//05.04.99
//Umstrukturierung, Aufruf FB2 mit Multiinstanz-DB
//Lesen von numMagPlaceParam bei Neustart da Änderung Anzahl Par. in SW 5 (8)
//DB92 - DB94 entfallen da Aufruf FB2 mit Multiiinstanz-DB
//neue Fkt: TNr_write=1, Vorgabe TNummer in TNr_FB2 von extern
//


FUNCTION_BLOCK FB 91
TITLE = LE_SUCH
// Fehler-Nr. in Ausgangsparameter State:
// 1 = Fehler FB2 interne T-Nummer lesen
// 2 = Kein Werkzeug in LocNr_ZW vorhanden
// 3 = Fehler FB4 PI-Dienst TMFDPL
// 4 = Fehler FB2 Rückgabeparameter lesen
// 5 = Leerplatzsucheauftrag mit Fehler beendet
//     Rückmeldung PI-Dienst von Variablen
// 6 = Schrittnummer unzulaessig
// 7 = Fehler Variable numPlaceParams lesen
//     -> Neustart erforderlich
// 8 = Fehler FB4 PI-Dienst MMCSEM
VERSION : 2.0

VAR_INPUT
    Start: Bool; // Start Leerplatz suchen für WZ in Zwischensp. mit pos.Flanke
    MagNr_ZW: Int; // Magazin-Nr. Zwischenspeicher
    LocNr_ZW: Int; // Platz-Nr. Zwischenspeicher
    MagNr: Int; // Magazin-Nr. der Leerplatzsuche
END_VAR

VAR_OUTPUT
    Activ:	Bool; // Baustein aktiv, Leerplatzsuche läuft
    Done: Bool; // Leerplatz gefunden
    Error: Bool; // Fehler
    State: Word; // Fehler-Nummer
    MagNr_Empty: Int; // Magazin-Nr. Leerplatz
    LocNr_Empty: Int; // Platz-Nr. Leerplatz
END_VAR

VAR
    TOANr: Byte:=b#16#1; // TOA-Bereich
    TNr_FB2: Int; // T-Nummer Magazinplatz
    TNr_write: Bool:=False; // Status=1:T-Nummer von Anwender versorgt
    MMCSEM: Bool:=False; // Status=1:Semaphoren nicht setzen
    numMagPlaceParams: Word; // Anzahl Parameter eines Magzinplatzes
    numPlacePar_read: Bool; //Variable nummagplaceparams lesen nach Neustart
    numPlacePar_Error: Bool; // Fehler bei Variable nummagplaceparams lesen
    numPlacePar_ok: Bool; // Variable numMagPlaceParams gelesen ohne Fehler
    HM_Fehler: Bool;
    Schrittregister : BYTE ;
    StateFB2_TNrGesp: Word; // Ausgang State FB2 T-Nr. lesen gespeichert
    StateFB2_ParGesp: Word; // Ausgang State FB2 Parameter lesen gespeichert
    StateFB4_Gesp:Word; // Ausgang State FB4 PI-Dienst Leerplatz suchen gespeichert
    BeZustdMag: Word; // Bereich Befehlszustand des Magazins bei Par. lesen
    MagNrLeerplatz: Word; // Bereich Magazin-Nummer Leerplatz bei Par.lesen
    PlNrLeerplatz: Word; // Bereich Platz-Nummer Leerplatz bei Par. lesen
    Value: Word; // Semaphore Value
    Zaehler: Int; // Zähler für Zeitüberwachung State 3 bei
    GET_FB2 : FB 2;
    PI_Dienste_FB4 : FB 4;
END_VAR
VAR_TEMP
    Error_FB2: Bool; // Error FB2
    NDR_FB2: Bool; // Auftrag beendet FB2
    Error_FB4: Bool; // Error FB4
    Done_FB4: Bool; // Auftrag beendet FB4
    LocLine: Word; // Zeilenadresse Log. T-Nr. lesen
    Column_FB2: Word; // Spaltenadresse FB2
    State_FB2: Word; // Fehler-Nr. FB2 T-Nr. lesen
    State_FB4: Word; // Fehler-Nr. FB4
    TOA: Int; // Eingang Unit FB4 PI-Dienst Leerplatz suchen
    TNr: Word; // Eingang WVar1 FB4 PI-Dienst Leerplatz suchen
    PlNrWohin: Word; // Eingang WVar2 FB4 PI-Dienst Leerplatz suchen
    MagNrWohin: Word; // Eingang WVar3 FB4 PI-Dienst Leerplatz suchen
    PlNr_Bez:  Word; // Eingang WVar4 FB4 PI-Dienst Leerplats suchen
    MagNr_Bez: Word; // Eingang WVar5 FB4 PI-Dienst Leerplats suchen
END_VAR

BEGIN
     UN	DB8.DBX45.0;
     SPB 	ANF1;		// Neustart ? Nein ->
     CALL	#GET_FB2 (
      	Req				:= FALSE);
     CALL	#PI_Dienste_FB4  (
		Req				:= FALSE);
	SET;
      R	numPlacePar_Error;
 	S	numPlacePar_read;
	R      numPlacePar_ok;
	SPA	LOEP;
ANF1:UN	numPlacePar_read;
     SPB	ANF2;
     call #GET_FB2 ( // -- Anzahl Parameter eines Magazinplatz lesen --
     Req:=TRUE, // Variable lesen
     NumVar:= 1, // Anzahl der zu lesenden Variablen
     Addr1:=WZV_VAR.N_Y_numMagPlaceParams_27, // Variable numMagPlaceParams
     Error:=#Error_FB2, // NC_VAR lesen beendet mit Fehler
     NDR:=#NDR_FB2, // NC_VAR lesen beendet ohne Fehler
     State:=#State_FB2, // Fehler-Nummer bei Error = 1
     RD1:=numMagPlaceParams); // Wert in numMagPlaceParams
     UN    #NDR_FB2; // Lesen beendet ohne Fehler
     UN    #Error_FB2; // Lesen beendet mit Fehler
     SPB   ENDE; // Lesen beendet ? Nein ->
     call #GET_FB2 ( // FB2 freigeben
     Req:=False);
     UN    #Error_FB2;
     R     numPlacePar_read;
     S     numPlacePar_ok;
     SPB   ENDE; // Lesen beendet mit Fehler ? Nein ->
     L     6;
     L     #State_FB2;
     ==I;
     SPB   ENDE; // FIFO voll -> Lesen wiederholen
     S     numPlacePar_Error;
     R     numPlacePar_read;
     T     StateFB2_TNrGesp; // Fehlernummer speichern
     SPA   ENDE;
ANF2:U   Start;
     SPB ANF;
LOEP:R    Done; // Ausgangsparameter Done nur 1 PLC-Zyklus
     R    Error; // Ausgangsparameter Error nur 1 PLC-Zyklus
     R    Activ;
     L    0;
     T    State; // Fehler-Nr. = 0
     SPA  ENDE;
ANF: U    Activ;
     SPB  SPRG; // Baustein aktiv ? Ja ->
     U   numPlacePar_Error;
     ON  numPlacePar_ok;
     L	7;
     SPB  FEHL; // Fehler bei Variable numMagPlaceParams lesen ->
     S    Activ; // Hilfsvariable vorbesetzen
     R    Done;
     R    Error;
     R    HM_Fehler;
     L    0;
     T    Zaehler;
     T    State; // Fehler-Nr. = 0
     T    MagNr_Empty;
     T    LocNr_Empty;
     T    Schrittregister;
SPRG:L    Schrittregister;
     SPL  FEHS; // Sprungverteiler
     SPA  SR1; // T-Nr. lesen
     SPA  SR2; // Semaphore setzen
     SPA  SR3; // Start PI-Dienst Leerplatz suchen
     SPA  SR4; // Rückgabeparameter lesen
     SPA  SR5; // Semaphore freigeben
FEHS:L 6;
     SPA  FEHL;
SR1: U    TNr_write;
     SPB  QFEH; // T-Nummer von Anwender -> keine TNr lesen
     L    MagNr_ZW; // ----Schritt 1: T-Nr. lesen --------------------
     T    Column_FB2; // Spalte Addr1 = Magazin-Nummer
     L    LocNr_ZW; // Platz-Nr. Zwischenspeicher
     +    -1;
     L    numMagPlaceParams; // Anzahl Parameter pro MagPlatz
     *I; // (PlatzNr.-1)*numMagPlaceParams+Parameter-Nr.
     +    3;
      T #LocLine; // Zeile Addr1 = T-Nr. von Platz 3
     call #GET_FB2 ( // -- Magazinplatzdaten lesen --
     Req:=TRUE, // Variable lesen
     NumVar:= 1, // Anzahl der zu lesenden Variablen
     Addr1:=WZV_VAR.T0_TP_placeData0_0, // T-Nummer von WZ in Zwischenspeicher
     Unit1:=TOANr, // Bereich = TOA 1
     Line1:=#LocLine, // Zeilenadresse
     Column1:=#Column_FB2, // Spaltenadresse
     Error:=#Error_FB2, // NC_VAR lesen beendet mit Fehler
     NDR:=#NDR_FB2, // NC_VAR lesen beendet ohne Fehler
     State:=#State_FB2, // Fehler-Nummer bei Error = 1
     RD1:=TNr_FB2); // Zielbereich für T-Nummer = TNr_FB2
     UN    #NDR_FB2; // Lesen beendet ohne Fehler
     UN    #Error_FB2; // Lesen beendet mit Fehler
     SPB   ENDE; // Lesen beendet ? Nein ->
     call #GET_FB2 ( // FB2 freigeben
     Req:=False);
     UN    #Error_FB2;
     SPB   QFEH; // Lesen beendet mit Fehler ? Nein ->
     L	6;
     L	#State_FB2;
     ==I;
     SPB	ENDE;
     T StateFB2_TNrGesp; // Fehlernummer speichern
     L     1; // Fehler-Nummer FB 91 = 1
     SPA   FEHL;
QFEH:L     TNr_FB2;	// logische T-Nummer von WZ in Zwischenspeicher
     L     0;
     ==I;
     L     2;
     SPB   FEHL; // T-Nr. in Zwischensp. = 0 ? -> Kein Leerplatz suchen
     U     MMCSEM;
     SPB  SR3A; // Semaphoren nicht setzen ->
     L     1;
     T     Schrittregister;
     T     Value;
SR2: L     TOANr;
     T     #TOA;
     CAll  #PI_Dienste_FB4 ( // -- PI-Dienst Semaphoren starten --
     Req:=TRUE, // Start PI-Dienst
     PIService:=PI.MMCSEM, // PI-Dienst Leerplatz suchen
     Unit:=#TOA, // TO-Nummer
     WVar1:=w#16#2, // FunctionNumber =2
     WVar2:=Value, // Semaphore Value
     Error:=#Error_FB4,
     Done:=#Done_FB4,
     State:=#State_FB4);
     UN    #Error_FB4;
     UN    #Done_FB4;
     SPB   ENDE;	// Leerplatzsuche beendet ? Nein ->
     CALL #PI_Dienste_FB4 ( // -- PI-Dienst Leerplatz suchen  beenden --
     Req:=False); // Start PI-Dienst
     UN    #Error_FB4;
     SPB   QFE1; // Leerplatzsuche beendet mit Fehler ? Nein ->
     L     #State_FB4;
     T     StateFB4_Gesp; // Fehler-Nummer FB 4 speichern
     L     3;
     <>I;
     L     8; // Fehler-Nummer FB 91 = 8
     SPB   FEHL;
     L     1;
     L     Schrittregister;
     <>I;
     L     8;
     SPB   FEHL; // Fehler bei Abwahl Semaphore
     L     Zaehler;
     +     1;
     T     Zaehler;
     L     300;
     >=I;
     L     8;
     SPB   FEHL; // Wartezeit ´überschritten ->
     SPA   ENDE; // Semaphore setzen wiederholen bis kein Fehler kommt
QFE1:U     HM_Fehler;
     SPB   FEH2;
     L     4;
     L     Schrittregister;
     ==I;
     SPB   SR5E; // Schritt 5 aktiv ? ->
SR3A:L     2; // --- Schritt 3: Start PI-Dienst Leerplatz suchen
     T     Schrittregister;
SR3: L     TOANr;
     T     #TOA; // TO-Nummer
     L     TNr_FB2;
     T     #TNr; // T-Nummer
     L     -1;
     T     #PlNrWohin; // Platz-Nummer Ziel = -1 -> nach Platznummer suchen
     L     MagNr;
     T     #MagNrWohin;	// Magazinnummer = 1
     L     LocNr_ZW;
     T     #PlNr_Bez;	// Platz-Nummer Wz für Leerplatzsuche
     L     MagNr_ZW;
     T     #MagNr_Bez;	// Magazin-Nummer Wz für Leerplatzsuche
     CAll  #PI_Dienste_FB4 ( // -- PI-Dienst Leerplatz suchen starten --
     Req:=TRUE, // Start PI-Dienst
     PIService:=PI.TMFDPL, // PI-Dienst Leerplatz suchen
     Unit:=#TOA, // TO-Nummer
     WVar1:=#TNr, // logische T-Nummer
     WVar2:=#PlNrWohin, // Platz-Nummer Ziel
     WVar3:=#MagNrWohin, // Magazin-Nummer Ziel
     WVar4:=#PlNr_Bez, // Platz-Nummer Werkzeug
     WVar5:=#MagNr_Bez, // Magazin-Nummer Werkzeug
     Error:=#Error_FB4,
     Done:=#Done_FB4,
     State:=#State_FB4);
     UN    #Error_FB4;
     UN    #Done_FB4;
     SPB   ENDE;	// Leerplatzsuche beendet ? Nein ->
     CALL #PI_Dienste_FB4 ( // -- PI-Dienst Leerplatz suchen  beenden --
     Req:=False); // Start PI-Dienst
     UN    #Error_FB4;
     SPB   QFE2; // Leerplatzsuche beendet mit Fehler ? Nein ->
     L     #State_FB4;
     T     StateFB4_Gesp; // Fehler-Nummer FB 4 speichern
     L     3; // Fehler-Nummer FB 91 = 3
     SPA   FEH1;
QFE2:L     3; // --- Schritt 4: Rückmeldungen über Variblendienst lesen
     T     Schrittregister;
SR4: call #GET_FB2 ( // Variable Rückgabeparameter lesen
     Req:=TRUE,
     NumVar:= 3,
     Addr1:=WZV_VAR.T0_TMC_magCBCmd1_0, // Befehlszustand des Magazins
     Unit1:=TOANr, // Bereich = TOA
     Column1:=w#16#8, // Spaltenadresse
     Addr2:=WZV_VAR.T0_TMC_magCBCmd1_0, // Magazin-Nummer Leerplatz
     Unit2:=TOANr, // Bereich = TOA
     Column2:=w#16#9, // Spaltenadresse
     Addr3:=WZV_VAR.T0_TMC_magCBCmd1_0, // Platz-Nummer Leerplatz
     Unit3:=TOANr, // Bereich = TOA
     Column3:=w#16#A, // Spaltenadresse
     Error:=#Error_FB2,
     NDR:=#NDR_FB2,
     State:=#State_FB2,
     RD1:=BeZustdMag,	// Bereich Befehlszustand des Magazins
     RD2:=MagNrLeerplatz, // Bereich Magazin-Nummer Leerplatz
     RD3:=PlNrLeerplatz); // Bereich Platz-Nummer Leerplatz
     UN    #Error_FB2;
     UN    #NDR_FB2;
     SPB   ENDE; //  Rückgabeparameter lesen beendet ? nein ->
     call #GET_FB2 ( // Variable Rückgabeparameter lesen beenden
     Req:=FALSE);
     UN    #Error_FB2;
     SPB   QFE3; // Par. Lesen mit Fehler beendet ? Nein ->
     L	6;
     L     #State_FB2;
     ==I;
     SPB	ENDE;
     T     StateFB2_ParGesp; // Fehler-Nr. FB2 speichern
     L     4; // Fehler-Nr. FB91 = 4
FEH1:T     State;
     U     MMCSEM;
     SPB   FEHL; // Ohne Semaphoren ->
     S     HM_Fehler;
     SPA   SR41;
QFE3:L     3;
     L     BeZustdMag;
     <>I;
     SPB   Weit; // Ende Korrekt ? Nein ->
     U     MMCSEM;
     SPB   SR5E; // Ohne Semaphoren ->
SR41:L     4; // Schritt 5 anwählen
     T     Schrittregister;
     L     0; // Semaphore freigeben
     T     Value;
     U     HM_Fehler;
     SPB   ENDE;
SR5: SPA   SR2; // Schritt 5: Semaphore freigeben
SR5E:S     Done;
     R     Activ;
     L     MagNrLeerplatz; // Magazin-Nummer Leerplatz
     T     MagNr_Empty;
     L     PlNrLeerplatz; // Platz-Nummer Leerplatz
     T     LocNr_Empty;
     L     0;
     T     Schrittregister; // Schrittregister auf Anfang
     SPA   ENDE;
Weit:L     4;
     <>I;
     SPB   ENDE; // Leerplatzsuche beendet mit Fehler ? Nein ->
     L     5;    // Ja
     S     HM_Fehler;
     SPA   SR41;
FEHL:T     State; // Fehler-Nummer FB91 ausgeben
FEH2:S     Error;
     R     Activ;
     L     0;
     T     Schrittregister; // Schrittregister auf Anfang
ENDE:NOP   0
END_FUNCTION_BLOCK

DATA_BLOCK db 91

        VERSION: 2.0

fb 91
Begin
END_DATA_BLOCK

